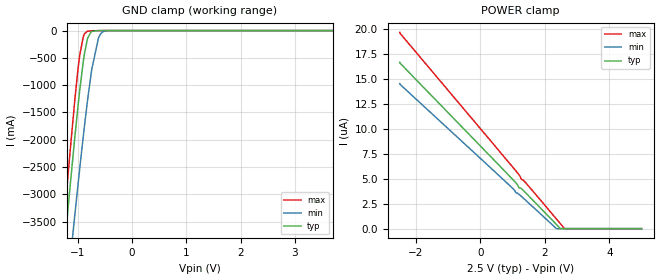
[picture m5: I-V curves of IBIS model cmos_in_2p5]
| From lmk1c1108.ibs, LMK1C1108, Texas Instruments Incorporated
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[Model]   cmos_in_2p5
Model_type   Input
Vinl = 0.75
Vinh = 1.75
|   typ   min   max
C_comp   7.053pF   6.6828pF   7.558pF
[Voltage Range]   2.5   2.375   2.625
[Temperature Range]   25   150   -40
[Power Clamp Reference]   2.5   2.375   2.625
[GND Clamp Reference]   0   0   0
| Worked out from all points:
|   GND clamp passes 1 mA (typ) near -0.62 V on its own axis
[GND Clamp]
|   Voltage   I(typ)   I(min)   I(max)
-2.5V     -17.66A    -16.51A    -19.55A
-1.375V   -5.426A    -6.588A    -4.973A
-1.173V   -3.215A    -4.559A    -2.596A
-1.143V   -2.896A    -4.263A    -2.256A
-1.06V    -2.04A     -3.461A    -1.356A
-962.5mV  -1.102A    -2.54A     -459.1mA
-895mV    -560mA     -1.93A     -106.4mA
-820mV    -157.3mA   -1.298A    -13.13mA
-737.5mV  -15.62mA   -700.8mA   -3.775mA
-617.5mV  -442.5uA   -142mA     -472.6uA
-497.5mV  -19.8uA    -9.13mA    -21.3uA
5V        0A         0A         0A
[POWER Clamp]
|   Voltage   I(typ)   I(min)   I(max)
-2.5V     16.66uA    14.53uA    19.66uA
1.01V     4.902uA    4.008uA    6.132uA
1.107V    4.565uA    3.586uA    5.753uA
1.205V    4.072uA    3.421uA    5.358uA
1.272V    4.001uA    3.229uA    4.951uA
1.333V    3.817uA    3.054uA    4.845uA
1.43V     3.5uA      2.767uA    4.507uA
2.353V    434.3nA    13.49nA    987.5nA
2.48V     8.302nA    0A         497.6nA
2.607V    0A         0A         7.609nA
5V        0A         0A         0A
